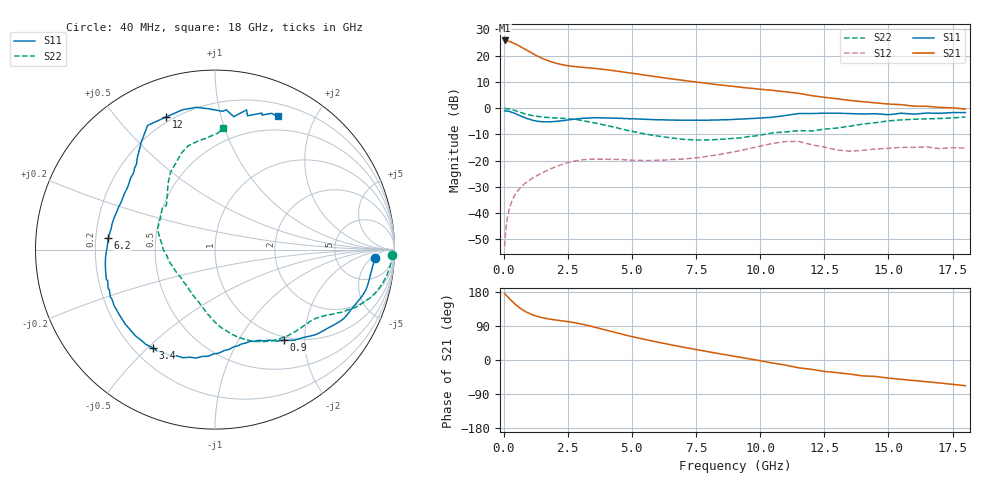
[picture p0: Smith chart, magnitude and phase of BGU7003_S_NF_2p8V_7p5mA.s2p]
!	Filename:	P:\Prog\Test\Noise\ATS_data\Testdata_Net\BGU7002	BGU7003	RN20082092\BGU7003_B1_high	freq_bias	loop_2.88V6.82mA_D.s2p
!	Date/Time:	Tue	16-Sep-08	9:24:25
!	BGU7003_B1_high	freq_bias	loop
!	bias	mode	1:00	Vout=	2.879	"V,"	Iout=	6.885	"mA,"	Vin=	3.105	"V,"	Iin=	0.661	mA
!	Date/time	Mon	Aug	11	2:51:14	2008
!	Device	data	file	deembeded	for	feedlines	and	parallel
!	Original	file:	\BGU7002	BGU7003	RN20082092\BGU7003_B1_high	freq_bias	loop_2.88V6.82mA_R.s2p
!	Feed-files:	PR029V01_high	"frequency_140808_Feed1.s2p,"	PR029V01_high	frequency_140808_Feed2.s2p
!	Parallel-file:	PR029V01_high	frequency_140808_Par.s2p
#	MHz	S	MA	R	50
!	Freq-MHz	S11-mag	S11-arg	S21-mag	S21-arg	S12-mag	S12-arg	S22-mag	S22-arg
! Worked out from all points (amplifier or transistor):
!   152 points, 40 MHz to 18 GHz, reference 50 ohm
!   highest |S21| = 25.8 dB at 40 MHz (marker M1)
!   |S21| within 3 dB of that: start of sweep to 769.7 MHz
!   unconditionally stable (mu >= 1): nowhere
!   at 290 MHz: K = 0.24, MSG = 30.7 dB, |S12| = -36.3 dB
!   at 2.05 GHz: K = 0.57, MSG = 19.7 dB, |S12| = -22.2 dB
!   at 18 GHz: K = 0.66, MSG = 7.4 dB, |S12| = -15.3 dB
!   lowest NFmin = 0.52 dB at 400 MHz
!   S11 on the Smith chart (normalised r, x): 40 MHz: 14, -6; 900 MHz: 0.94, -1.60; 3.4 GHz: 0.27, -0.52; 6.2 GHz: 0.25, +0.05; 12 GHz: 0.18, +0.68; 18 GHz: 0.33, +1.52
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40  0.891 -2.9  19.39 175.3  0.00235 65.6  0.9873 -1.7
140  0.876 -10.7  19.03 168.3  0.00765 77.8  0.9768 -6.3
240  0.8569 -18.0  18.48 160.9  0.01284 76.5  0.9565 -10.6
310  0.8318 -23.0  17.94 156.2  0.01625 74.8  0.9392 -13.3
440  0.793 -31.2  16.87 147.9  0.0222 71.4  0.8973 -17.9
550  0.7493 -37.7  15.79 141.5  0.02665 69.0  0.8628 -21.0
650  0.7153 -42.4  14.85 136.4  0.03044 67.1  0.8295 -23.4
900  0.6349 -52.6  12.6 126.2  0.03889 63.6  0.7619 -27.6
1100  0.5906 -58.7  11.09 120.0  0.0453 61.7  0.7228 -30.1
1250  0.5727 -62.5  10.17 116.4  0.05029 60.3  0.7025 -31.9
1650  0.5484 -71.8  8.284 109.6  0.06366 56.6  0.6673 -36.5
2350  0.579 -89.4  6.591 102.7  0.08676 47.0  0.6328 -47.3
3100  0.6408 -112.9  5.971 94.0  0.104 33.4  0.577 -63.1
3400  0.6481 -122.5  5.775 89.3  0.1061 28.5  0.5419 -69.1
4700  0.63 -159.1  4.83 66.6  0.1034 15.9  0.3883 -92.2
6200  0.5981 173.7  3.794 44.4  0.1019 16.6  0.2847 -114.5
7400  0.587 157.7  3.175 28.8  0.1114 18.8  0.248 -136.9
9200  0.6164 139.7  2.51 7.5  0.1544 18.8  0.2693 -172.2
12000  0.7877 110.1  1.727 -24.6  0.2009 -26.9  0.3662 137.7
12500  0.7996 103.2  1.605 -30.1  0.1812 -31.2  0.3977 132.1
15500  0.798 77.3  1.161 -51.0  0.1786 -33.1  0.5973 104.5
18000  0.8206 64.9  0.9576 -67.9  0.1726 -46.4  0.678 86.1
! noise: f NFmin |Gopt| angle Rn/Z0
400  0.522  0.303  9.46  0.132
1000  0.631  0.295  25.08  0.145
1500  0.722  0.289  38.09  0.151
1700  0.758  0.288  43.3  0.152
2200  0.849  0.285  56.32  0.151
3000  0.994  0.283  77.14  0.144
4400  1.249  0.291  113.6  0.119
5800  1.503  0.311  150  0.094
8000  1.902  0.369  -161.4  0.093
1.2e+04  2.629  0.553  -122  0.393
